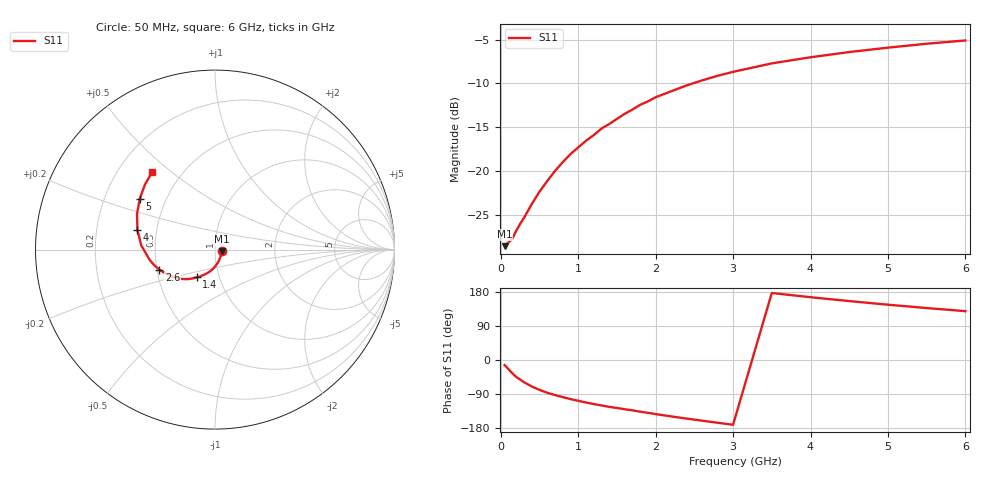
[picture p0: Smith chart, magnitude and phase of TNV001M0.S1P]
! SIEMENS Discrete & RF Semiconductors
! BAS70-07W
! Si Schottky Diode in SOT343
! IF = 1 mA
! S-Parameters:  February  1997
# GHz  S  MA  R  50
!  f  S11
! GHz  MAG  ANG
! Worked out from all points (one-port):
!   34 points, 50 MHz to 6 GHz, reference 50 ohm
!   lowest |S11| = -28.6 dB at 50 MHz (marker M1), VSWR 1.08, Z = 53.7 - j0.929 ohm
!   |S11| at or under -10 dB: start of sweep to 2.48 GHz
!   S11 on the Smith chart (normalised r, x): 50 MHz: 1.07, -0.02; 1.4 GHz: 0.78, -0.25; 2.6 GHz: 0.52, -0.13; 4 GHz: 0.39, +0.11; 5 GHz: 0.36, +0.27; 6 GHz: 0.34, +0.43
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0.05  0.03723 -13.4
0.15  0.04111 -35.2
0.2  0.04556 -44.8
0.25  0.04984 -51.5
0.3  0.05399 -58.6
0.4  0.06469 -69.8
0.5  0.07615 -78.9
0.7  0.1 -92.5
0.8  0.1122 -97.9
0.9  0.1248 -103.1
1.1  0.1488 -112.1
1.2  0.1602 -116.2
1.3  0.1746 -119.8
1.4  0.1853 -123.6
1.6  0.212 -130.0
1.7  0.2242 -132.8
1.8  0.2386 -136.4
1.9  0.2495 -139.3
2  0.2637 -142.7
2.4  0.308 -154.6
2.6  0.329 -160.1
3  0.3681 -170.9
3.5  0.4115 176.8
4  0.4459 165.7
4.5  0.4777 155.5
5  0.506 145.9
5.5  0.5327 137.1
6  0.5562 128.9
